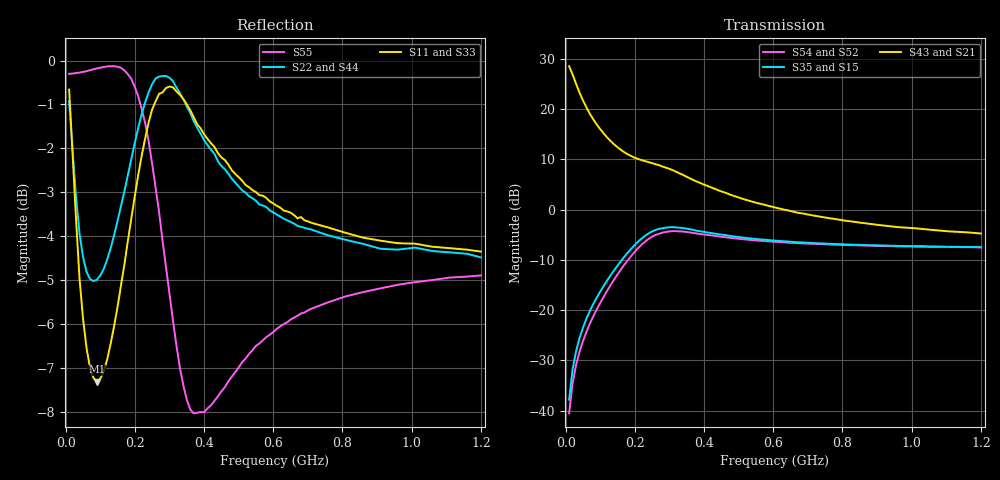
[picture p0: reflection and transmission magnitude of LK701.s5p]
! Date: Wed May 20 11:17:12 1998
!  POLYFET RF DEVICES
!  LP701/LK701
!  28Vdc		200ma
!AWR Design Environment (2053) Wed Feb 04 14:51:27 2004
!freq-unit  param-type  data-format  keyword  impedance-ohms
# MHz  S  MA  R  50
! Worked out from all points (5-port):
!   120 points, 10 MHz to 1.2 GHz, reference 50 ohm
!   strongest paths, dB at 10 MHz, 310 MHz, 610 MHz, 910 MHz, 1.2 GHz:
!     S43: 28.5, 7.8, 0.3, -3.1, -4.8
!     S21: 28.5, 7.8, 0.3, -3.1, -4.8
!     S35: -37.8, -3.5, -6.2, -7.1, -7.5
!     S15: -37.8, -3.5, -6.2, -7.1, -7.5
!     S54: -40.5, -4.3, -6.4, -7.2, -7.5
!     S52: -40.5, -4.3, -6.4, -7.2, -7.5
!   lowest |S11| = -7.3 dB at 90 MHz (marker M1), VSWR 2.51, Z = 51.2 - j48.3 ohm
!   |S11| at or under -10 dB: nowhere
